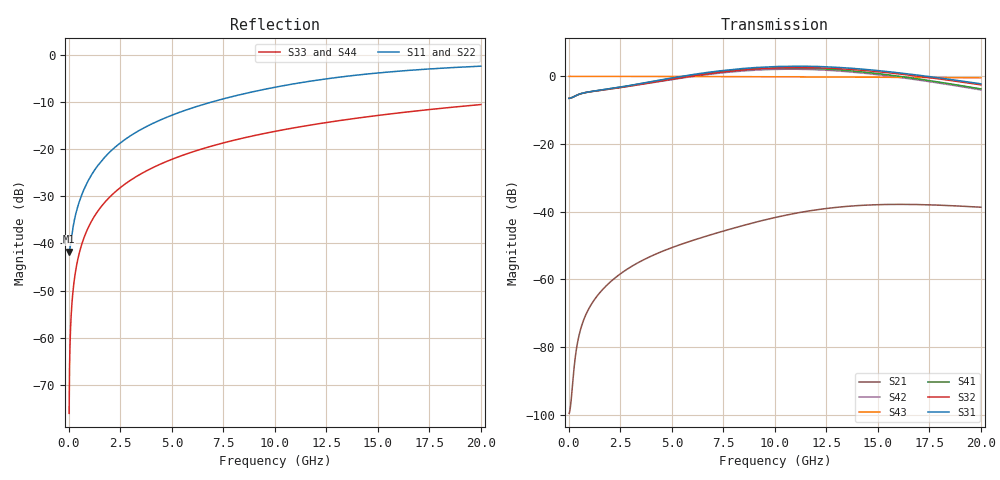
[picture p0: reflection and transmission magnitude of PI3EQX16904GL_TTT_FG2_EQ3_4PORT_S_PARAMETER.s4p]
! NPort=4 DATA=2000 NOISE=0 GROUPDELAY=0 COMPLEX_DATAFORMAT=POLAR
! NumOfBlock=1 NumOfParam=0
! .MODEL Smodel S TSTONEFILE=PI3EQX16904GL_TTT_FG2_EQ3_4PORT_S_PARAMETER.s4p TYPE=S
!  -- The above .MODEL line can be used for the S element in the netlist.
! The s parameter is extracted from the linear redriver, it is not bi-directional; only s(4,1)s(4,2) and s(3,1)s(3,2)
! should be the insertion loss
!Port definition:
!Port1 = input+
!Port2 = input-
!Port3 = output+
!Port4 = output-
# Hz S MA R  50
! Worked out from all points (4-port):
!   2000 points, 10 MHz to 20 GHz, reference 50 ohm
!   strongest paths, dB at 10 MHz, 5.01 GHz, 10.01 GHz, 15.01 GHz, 20 GHz:
!     S31: -6.5, -0.4, 2.9, 1.7, -2.2
!     S32: -6.5, -0.8, 2.5, 1.4, -2.5
!     S41: -6.5, -0.6, 2.5, 0.8, -3.7
!     S43: 0.0, 0.0, -0.1, -0.3, -0.4
!     S42: -6.5, -0.9, 2.1, 0.5, -4.0
!     S21: -99.6, -50.6, -41.7, -37.9, -38.7
!   lowest |S11| = -41.7 dB at 10 MHz (marker M1), VSWR 1.02, Z = 49.2 - j0.0603 ohm
!   |S11| at or under -10 dB: start of sweep to 6.903 GHz
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1e7  0.008182 -175.7  1.05e-05 7.6  0 0.0  0 0.0
     1.05e-05 7.6  0.008182 -175.7  0 0.0  0 0.0
     0.4743 0.2  0.4743 -179.8  0.0001571 -90.0  1 -0.0
     0.4743 -179.8  0.4743 0.2  1 -0.0  0.0001571 -90.0
4e8  0.02342 -118.9  0.0001085 117.3  0 0.0  0 0.0
     0.0001085 117.2  0.02342 -118.9  0 0.0  0 0.0
     0.5303 6.1  0.5296 -174.3  0.006283 -90.4  1 -0.4
     0.5302 -174.7  0.5295 5.0  1 -0.4  0.006283 -90.4
1.67e9  0.07925 -102.6  0.0007266 104.9  0 0.0  0 0.0
        0.0007266 104.8  0.07926 -102.7  0 0.0  0 0.0
        0.6351 -0.0  0.6299 178.9  0.02622 -91.6  0.9996 -1.5
        0.6342 177.0  0.629 -4.1  0.9996 -1.5  0.02622 -91.6
6.18e9  0.2835 -105.4  0.003938 81.4  0 0.0  0 0.0
        0.003913 81.3  0.2834 -105.5  0 0.0  0 0.0
        1.084 -40.0  1.032 139.1  0.09658 -95.8  0.995 -5.5
        1.063 129.1  1.012 -51.9  0.995 -5.5  0.09658 -95.8
1.015e10  0.4623 -113.2  0.008483 54.3  0 0.0  0 0.0
          0.008396 54.9  0.4614 -113.3  0 0.0  0 0.0
          1.401 -99.4  1.337 80.8  0.1573 -99.4  0.9866 -9.0
          1.332 63.0  1.271 -116.9  0.9866 -9.0  0.1573 -99.4
1.427e10  0.6229 -123.4  0.01253 12.9  0 0.0  0 0.0
          0.01245 13.8  0.6216 -123.4  0 0.0  0 0.0
          1.279 -165.8  1.229 14.6  0.2183 -103.1  0.9739 -12.6
          1.163 -9.8  1.117 170.6  0.9739 -12.6  0.2183 -103.1
2e10  0.7633 -135.8  0.01171 -34.6  0 0.0  0 0.0
      0.01166 -33.3  0.7626 -135.7  0 0.0  0 0.0
      0.7755 114.8  0.7489 -64.7  0.2986 -108.1  0.9506 -17.4
      0.653 -97.1  0.6306 83.3  0.9506 -17.4  0.2986 -108.1
